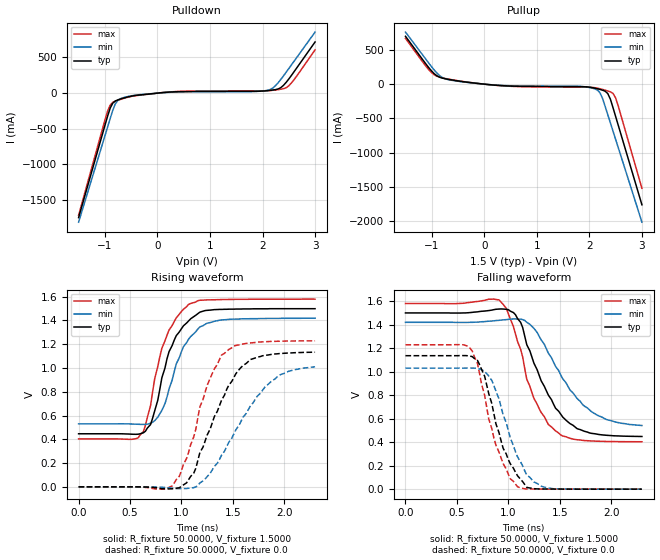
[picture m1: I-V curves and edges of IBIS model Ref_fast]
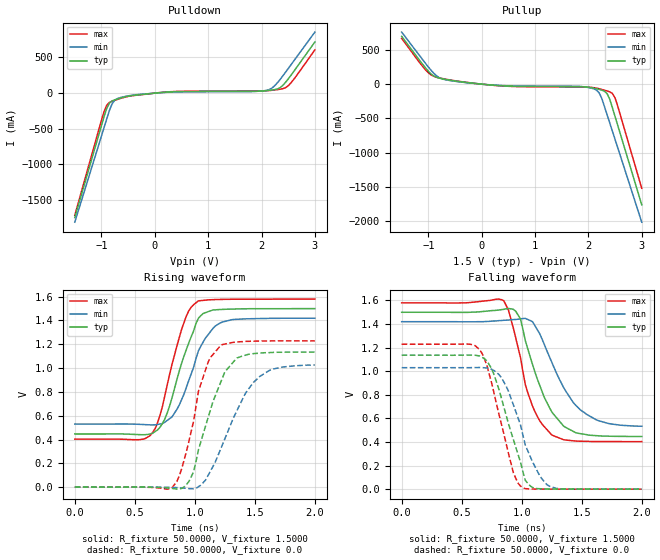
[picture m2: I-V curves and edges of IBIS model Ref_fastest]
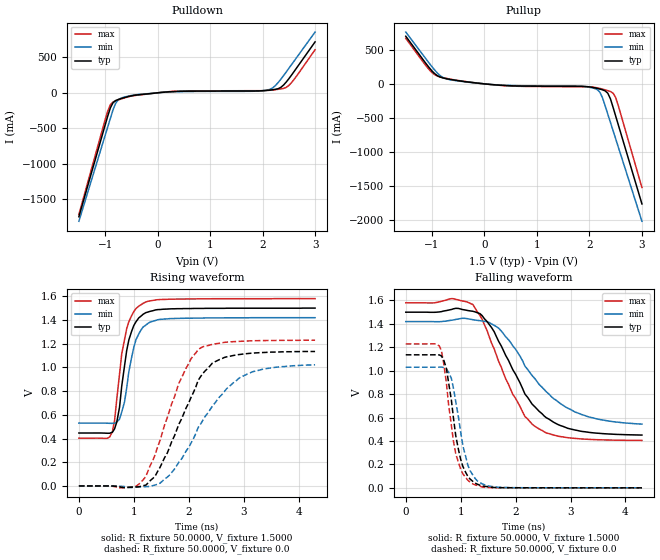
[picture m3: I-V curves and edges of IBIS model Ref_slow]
| Integrated Devices Technolgy, Inc
[IBIS Ver]   4.1
[File name]   9fgu0631.ibs
[File Rev]   1.0
|Rev history   1.0   original revision, 906 LP_HCSL updated for 1.5V operation, IH
[Date]   09 October, 2015
[Disclaimer] Integrated Device Technology, Inc. ("IDT") hereby grants the
   user of this ibis model a non-exclusive, nontransferable
   license to use this ibis model under the following terms. the
   user is granted this license only to use the ibis model and is
   not granted rights to sell, copy (except as needed to run the
   ibis model), rent, lease or sub-license the ibis model in
   whole or in part, or in modified form to anyone. the user may
   modify the ibis model to suit its specific applications, but
   rights to derivative works and such modifications shall belong
   to idt. this ibis model is provided on an as is" basis and idt
   makes absolutely no warranty with respect to the information
   contained herein. idt disclaims and customer waives all
   warranties, express and implied, including warranties of
   merchantability and fitness for a particular purpose. the
   entire risk as to quality and performance is with the user
   accordingly, in no event shall idt be liable for any direct or
   indirect damages, whether in contract or tort, including any
   lost profits or other incidental, consequential, exemplary, or
   punitive damages arising out of the use or application of the
   ibis model. further, idt reserves the right to make changes
   without notice to any product herein to improve reliability,
   function, or design. idt does not convey any license under
   patent rights or any other intellectual property rights,
   including those of third parties. idt is not obligated to
   provide maintenance or support for the licensed ibis model.
[Copyright]   Copyright 2012, Integrated Devices Technolgy, Inc. all rights
   reserved
[Component]   9fgu0631
[Manufacturer] Integrated Device Technology, Inc.
[Package]
|40-VFQFPN
|variable   typ   min   max
R_pkg   81.1m   62.2m   100.0m
L_pkg   6.7nH   4.9nH   8.5nH
C_pkg   0.53pF   0.21pF   0.85pF
[Pin] signal_name  model_name
1   vSS_EN_tri   IN
2   XIN/CLKIN_25   IN
3   X2   NC
4   VDDXTAL1.5   POWER
5   VDDREF1.5   POWER
6   vSADR/REF1.5   REF
7   NC   NC
8   GNDDIG   GND
9   SCLK_3.3   SCIN
10   SDATA_3.3   SCIN
11   VDDDIG1.5   POWER
12   VDDIO   POWER
13   vOE0#   IN
14   DIF0   LP_HCSL
15   DIF0#   LP_HCSL
16   VDD1.5   POWER
17   VDDIO   POWER
18   DIF1   LP_HCSL
19   DIF1#   LP_HCSL
20   NC   NC
21   vOE1#   IN
22   DIF2   LP_HCSL
23   DIF2#   LP_HCSL
24   vOE2#   IN
25   NC   NC
26   VDDA1.5   POWER
27   VDDIO   POWER
28   DIF3   LP_HCSL
29   DIF3#   LP_HCSL
30   vOE3#   IN
31   VDD1.5   POWER
32   VDDIO   POWER
33   DIF4   LP_HCSL
34   DIF4#   LP_HCSL
35   vOE4#   IN
36   DIF5   LP_HCSL
37   DIF5#   LP_HCSL
38   vOE5#   IN
39   VDDIO   POWER
40   ^CKPWRGD_PD   PD
41   ePAD   GND
[Diff Pin]  inv_pin  vdiff tdelay_typ tdelay_min  tdelay_max
14   15   NA   0   0   0
18   19   NA   0   0   0
22   23   NA   0   0   0
28   29   NA   0   0   0
33   34   NA   0   0   0
36   37   NA   0   0   0
[Model Selector] REF
Ref_fast amplitude 1.5, slew rate fast
Ref_fastest amplitude 1.5, slew rate fastest
Ref_slow amplitude 1.5, slew rate slow
Ref_slowest amplitude 1.5, slew rate slowest
[Model Selector] LP_HCSL
lphcsl_0v6_fast amplitude 0.6V, slew rate fast
lphcsl_0v6_slow amplitude 0.6V, slew rate slow
lphcsl_0v7_fast amplitude 0.7V, slew rate fast
lphcsl_0v7_slow amplitude 0.7V, slew rate slow
lphcsl_0v8_fast amplitude 0.8V, slew rate fast
lphcsl_0v8_slow amplitude 0.8V, slew rate slow
lphcsl_0v9_fast amplitude 0.9V, slew rate fast
lphcsl_0v9_slow amplitude 0.9V, slew rate slow
| Models and submodels in the file (15): Ref_fast (Output), Ref_fastest (Output), Ref_slow (Output), Ref_slowest (Output), lphcsl_0v6_fast (Output), lphcsl_0v6_slow (Output), lphcsl_0v7_fast (Output), lphcsl_0v7_slow (Output), lphcsl_0v8_fast (Output), lphcsl_0v8_slow (Output), lphcsl_0v9_fast (Output), lphcsl_0v9_slow (Output), IN (Input), SCIN (Input), PD (Input)
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[Model]  Ref_fast
Model_type Output
Polarity   Non-Inverting
Enable   Active-High
Vmeas =  0.9000V
Cref =   5.0000pF
Rref =   0.0
Vref =   0.9000V
C_comp   1.1000pF   1.0000pF   1.2000pF
[Temperature Range]   25.0000   75.0000   0.0
[Voltage Range]   1.5000V   1.4200V   1.5800V
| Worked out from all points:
|   slope of the pulldown table from 0 to 0.225 V, typ, clamps not added: 15.7 ohm
|   slope of the pullup table from 0 to 0.225 V, typ, clamps not added: 14.4 ohm
|   rising waveform, R_fixture 50.0000, V_fixture 1.5000: 20-80 % time 219ps typ, 227ps min, 214ps max; typ from 0.446 V to 1.5 V
|   rising waveform, R_fixture 50.0000, V_fixture 0.0: 20-80 % time 341ps typ, 434ps min, 263ps max; typ from 0 V to 1.13 V
|   falling waveform, R_fixture 50.0000, V_fixture 1.5000: 20-80 % time 330ps typ, 386ps min, 269ps max; typ from 1.5 V to 0.448 V
|   falling waveform, R_fixture 50.0000, V_fixture 0.0: 20-80 % time 229ps typ, 251ps min, 218ps max; typ from 1.14 V to 0 V
[Pulldown]
|Voltage   I(typ)   I(min)   I(max)
-1.5V     -1.745A    -1.809A    -1.713A
-950mV    -327.8mA   -480.1mA   -255.7mA
-900mV    -212.5mA   -359.3mA   -168.3mA
-850mV    -140.3mA   -241.1mA   -129.4mA
-750mV    -94.02mA   -98.51mA   -100.2mA
-450mV    -36.28mA   -31.57mA   -39.68mA
250mV     15.41mA    12.24mA    17.86mA
1.8V      25.49mA    21.55mA    29.47mA
2.15V     39.17mA    51.36mA    36.57mA
2.35V     77.57mA    193.2mA    55.3mA
2.5V      197.9mA    344.2mA    103.1mA
3V        716.8mA    855.6mA    606.3mA
[Pullup]
|Voltage   I(typ)   I(min)   I(max)
-1.5V     699.4mA    760.9mA    669.2mA
-1V       189.6mA    251.3mA    166.1mA
-900mV    121.4mA    161.2mA    115.6mA
-750mV    80mA       79.09mA    84.43mA
350mV     -22.11mA   -19.15mA   -24.57mA
1.8V      -36.31mA   -32.03mA   -41.75mA
2.15V     -66.71mA   -84.88mA   -58.33mA
2.25V     -87.88mA   -207.1mA   -76.93mA
2.35V     -137.7mA   -445.8mA   -99.43mA
2.45V     -344.5mA   -687.2mA   -135.9mA
2.5V      -473.4mA   -808mA     -201.5mA
3V        -1.763A    -2.017A    -1.522A
[Ramp]
| variable   typ   min   max
dV/dt_r  0.6798/0.3452n   0.6060/0.4303n   0.7374/0.2908n
dV/dt_f  0.6310/0.3319n   0.5270/0.3829n   0.7058/0.2936n
R_load = 50.0000
[Rising Waveform]
R_fixture= 50.0000
V_fixture= 1.5000
V_fixture_min= 1.4200
V_fixture_max= 1.5800
|time   V(typ)   V(min)   V(max)
0s        446.5mV    530.1mV    403.2mV
530ps     442.5mV    528.3mV    400.9mV
630ps     454.6mV    525.2mV    463.7mV
700ps     524.1mV    535.3mV    684.1mV
740ps     638.7mV    557.1mV    908.5mV
810ps     918.1mV    643.4mV    1.166V
950ps     1.272V     1.035V     1.422V
1.07ns    1.396V     1.242V     1.535V
1.37ns    1.493V     1.402V     1.575V
2.3ns     1.499V     1.419V     1.579V
[Rising Waveform]
R_fixture= 50.0000
V_fixture= 0.0
V_fixture_min= 0.0
V_fixture_max= 0.0
|time   V(typ)   V(min)   V(max)
0s        0V         0V         0V
910ps     -16.39mV   -11.25mV   7.954mV
980ps     -7.248mV   -15.17mV   88.84mV
1.14ns    156.1mV    -875uV     484.8mV
1.18ns    289.4mV    33.51mV    674.6mV
1.25ns    435.4mV    85.49mV    853.8mV
1.39ns    727.8mV    265.7mV    1.108V
1.58ns    1.005V     551.8mV    1.198V
1.95ns    1.121V     938.1mV    1.225V
2.3ns     1.133V     1.01V      1.229V
[Falling Waveform]
R_fixture= 50.0000
V_fixture= 1.5000
V_fixture_min= 1.4200
V_fixture_max= 1.5800
|time   V(typ)   V(min)   V(max)
0s        1.5V       1.42V      1.58V
910ps     1.533V     1.437V     1.611V
980ps     1.531V     1.443V     1.54V
1.12ns    1.42V      1.447V     1.191V
1.18ns    1.229V     1.42V      935.1mV
1.28ns    1.018V     1.335V     724.8mV
1.39ns    800.1mV    1.157V     549.9mV
1.56ns    588mV      907.6mV    446.1mV
1.81ns    475.1mV    659.1mV    410.3mV
2.3ns     448.4mV    541.7mV    403.6mV
[Falling Waveform]
R_fixture= 50.0000
V_fixture= 0.0
V_fixture_min= 0.0
V_fixture_max= 0.0
|time   V(typ)   V(min)   V(max)
0s        1.136V     1.03V      1.229V
630ps     1.132V     1.031V     1.198V
720ps     1.061V     1.023V     986.4mV
770ps     961.2mV    1.003V     799.1mV
840ps     728.3mV    925.3mV    515.6mV
950ps     348.1mV    632mV      217.3mV
1.09ns    114mV      275.1mV    20.31mV
1.18ns    14.99mV    120.1mV    1.832mV
1.35ns    1.542mV    17.53mV    713.8uV
2.3ns     16.86uV    43.33uV    1.931uV
[Model]  Ref_fastest
Model_type Output
Polarity   Non-Inverting
Enable   Active-High
Vmeas =  0.9000V
Cref =   5.0000pF
Rref =   0.0
Vref =   0.9000V
C_comp   1.1000pF   1.0000pF   1.2000pF
[Temperature Range]   25.0000   75.0000   0.0
[Voltage Range]   1.5000V   1.4200V   1.5800V
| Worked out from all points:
|   slope of the pulldown table from 0 to 0.225 V, typ, clamps not added: 15.7 ohm
|   slope of the pullup table from 0 to 0.225 V, typ, clamps not added: 14.4 ohm
|   rising waveform, R_fixture 50.0000, V_fixture 1.5000: 20-80 % time 199ps typ, 204ps min, 177ps max; typ from 0.446 V to 1.5 V
|   rising waveform, R_fixture 50.0000, V_fixture 0.0: 20-80 % time 214ps typ, 277ps min, 173ps max; typ from 0 V to 1.14 V
|   falling waveform, R_fixture 50.0000, V_fixture 1.5000: 20-80 % time 225ps typ, 269ps min, 184ps max; typ from 1.5 V to 0.447 V
|   falling waveform, R_fixture 50.0000, V_fixture 0.0: 20-80 % time 201ps typ, 211ps min, 177ps max; typ from 1.14 V to 0 V
[Pulldown]
|Voltage   I(typ)   I(min)   I(max)
-1.5V     -1.745A    -1.809A    -1.713A
-950mV    -327.8mA   -480.1mA   -255.7mA
-900mV    -212.5mA   -359.3mA   -168.3mA
-850mV    -140.3mA   -241.1mA   -129.4mA
-750mV    -94.02mA   -98.51mA   -100.2mA
-450mV    -36.28mA   -31.57mA   -39.68mA
250mV     15.41mA    12.24mA    17.86mA
1.8V      25.49mA    21.55mA    29.47mA
2.15V     39.17mA    51.36mA    36.57mA
2.35V     77.57mA    193.2mA    55.3mA
2.5V      197.9mA    344.2mA    103.1mA
3V        716.8mA    855.6mA    606.3mA
[Pullup]
|Voltage   I(typ)   I(min)   I(max)
-1.5V     699.4mA    760.9mA    669.2mA
-1V       189.6mA    251.3mA    166.1mA
-900mV    121.4mA    161.2mA    115.6mA
-750mV    80mA       79.09mA    84.43mA
350mV     -22.11mA   -19.15mA   -24.57mA
1.8V      -36.31mA   -32.03mA   -41.75mA
2.15V     -66.71mA   -84.88mA   -58.33mA
2.25V     -87.88mA   -207.1mA   -76.93mA
2.35V     -137.7mA   -445.8mA   -99.43mA
2.45V     -344.5mA   -687.2mA   -135.9mA
2.5V      -473.4mA   -808mA     -201.5mA
3V        -1.763A    -2.017A    -1.522A
[Ramp]
| variable   typ   min   max
dV/dt_r  0.6810/0.2229n   0.6156/0.2774n   0.7374/0.1932n
dV/dt_f  0.6319/0.2282n   0.5320/0.2690n   0.7060/0.2043n
R_load = 50.0000
[Rising Waveform]
R_fixture= 50.0000
V_fixture= 1.5000
V_fixture_min= 1.4200
V_fixture_max= 1.5800
|time   V(typ)   V(min)   V(max)
0s        446.5mV    530.1mV    403.2mV
630ps     447mV      523.1mV    434.1mV
690ps     481.3mV    526.5mV    542.2mV
750ps     572.5mV    545.7mV    768mV
850ps     902.3mV    652.2mV    1.183V
950ps     1.213V     897.3mV    1.482V
1.03ns    1.419V     1.145V     1.565V
1.15ns    1.488V     1.332V     1.575V
1.23ns    1.493V     1.387V     1.577V
2ns       1.5V       1.419V     1.58V
[Rising Waveform]
R_fixture= 50.0000
V_fixture= 0.0
V_fixture_min= 0.0
V_fixture_max= 0.0
|time   V(typ)   V(min)   V(max)
0s        0V         0V         0V
810ps     -10.62mV   -2.241mV   -4.352mV
890ps     -10.75mV   -6.644mV   152.2mV
1.01ns    216.9mV    -9.648mV   681.3mV
1.13ns    648.7mV    134.3mV    1.089V
1.25ns    967.4mV    405.7mV    1.202V
1.35ns    1.085V     641.1mV    1.219V
1.49ns    1.122V     882mV      1.226V
1.62ns    1.13V      979.7mV    1.228V
2ns       1.135V     1.026V     1.229V
[Falling Waveform]
R_fixture= 50.0000
V_fixture= 1.5000
V_fixture_min= 1.4200
V_fixture_max= 1.5800
|time   V(typ)   V(min)   V(max)
0s        1.5V       1.42V      1.58V
850ps     1.525V     1.432V     1.599V
890ps     1.532V     1.434V     1.517V
990ps     1.443V     1.444V     1.116V
1.03ns    1.26V      1.448V     888.1mV
1.09ns    1.058V     1.42V      704.3mV
1.25ns    655.5mV    1.078V     460.1mV
1.49ns    470.3mV    670.9mV    406.6mV
1.72ns    449.3mV    557.6mV    403.6mV
2ns       446.8mV    533.3mV    403.3mV
[Falling Waveform]
R_fixture= 50.0000
V_fixture= 0.0
V_fixture_min= 0.0
V_fixture_max= 0.0
|time   V(typ)   V(min)   V(max)
0s        1.136V     1.03V      1.229V
570ps     1.137V     1.03V      1.229V
650ps     1.129V     1.032V     1.183V
750ps     1.021V     1.017V     898.6mV
830ps     775.7mV    947.7mV    555.6mV
930ps     423.1mV    716.8mV    141.6mV
1.01ns    147.3mV    458.1mV    10.69mV
1.09ns    14.41mV    232mV      1.504mV
1.23ns    1.161mV    25.5mV     376.5uV
2ns       -22.42uV   21.58uV    0V
[Model]  Ref_slow
Model_type Output
Polarity   Non-Inverting
Enable   Active-High
Vmeas =  0.9000V
Cref =   5.0000pF
Rref =   0.0
Vref =   0.9000V
C_comp   1.1000pF   1.0000pF   1.2000pF
[Temperature Range]   25.0000   75.0000   0.0
[Voltage Range]   1.5000V   1.4200V   1.5800V
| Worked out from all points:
|   slope of the pulldown table from 0 to 0.225 V, typ, clamps not added: 15.7 ohm
|   slope of the pullup table from 0 to 0.225 V, typ, clamps not added: 14.4 ohm
|   rising waveform, R_fixture 50.0000, V_fixture 1.5000: 20-80 % time 212ps typ, 217ps min, 213ps max; typ from 0.446 V to 1.5 V
|   rising waveform, R_fixture 50.0000, V_fixture 0.0: 20-80 % time 647ps typ, 857ps min, 569ps max; typ from 0 V to 1.13 V
|   falling waveform, R_fixture 50.0000, V_fixture 1.5000: 20-80 % time 763ps typ, 912ps min, 658ps max; typ from 1.5 V to 0.451 V
|   falling waveform, R_fixture 50.0000, V_fixture 0.0: 20-80 % time 234ps typ, 246ps min, 226ps max; typ from 1.14 V to 0 V
[Pulldown]
|Voltage   I(typ)   I(min)   I(max)
-1.5V     -1.745A    -1.809A    -1.713A
-950mV    -327.8mA   -480.1mA   -255.7mA
-900mV    -212.5mA   -359.3mA   -168.3mA
-850mV    -140.3mA   -241.1mA   -129.4mA
-750mV    -94.02mA   -98.51mA   -100.2mA
-450mV    -36.28mA   -31.57mA   -39.68mA
250mV     15.41mA    12.24mA    17.86mA
1.8V      25.49mA    21.55mA    29.47mA
2.15V     39.17mA    51.36mA    36.57mA
2.35V     77.57mA    193.2mA    55.3mA
2.5V      197.9mA    344.2mA    103.1mA
3V        716.8mA    855.6mA    606.3mA
[Pullup]
|Voltage   I(typ)   I(min)   I(max)
-1.5V     699.4mA    760.9mA    669.2mA
-1V       189.6mA    251.3mA    166.1mA
-900mV    121.4mA    161.2mA    115.6mA
-750mV    80mA       79.09mA    84.43mA
350mV     -22.11mA   -19.15mA   -24.57mA
1.8V      -36.31mA   -32.03mA   -41.75mA
2.15V     -66.71mA   -84.88mA   -58.33mA
2.25V     -87.88mA   -207.1mA   -76.93mA
2.35V     -137.7mA   -445.8mA   -99.43mA
2.45V     -344.5mA   -687.2mA   -135.9mA
2.5V      -473.4mA   -808mA     -201.5mA
3V        -1.763A    -2.017A    -1.522A
[Ramp]
| variable   typ   min   max
dV/dt_r  0.6804/0.6793n   0.6132/0.8910n   0.7374/0.5687n
dV/dt_f  0.6296/0.7983n   0.5254/0.9479n   0.7052/0.6762n
R_load = 50.0000
[Rising Waveform]
R_fixture= 50.0000
V_fixture= 1.5000
V_fixture_min= 1.4200
V_fixture_max= 1.5800
|time   V(typ)   V(min)   V(max)
0s        446.5mV    530.1mV    403.2mV
610ps     452.9mV    527.7mV    456.5mV
650ps     482mV      529.1mV    552.8mV
740ps     662.8mV    563.9mV    942.7mV
780ps     841.5mV    623.1mV    1.113V
870ps     1.141V     826mV      1.326V
1ns       1.353V     1.169V     1.47V
1.17ns    1.448V     1.341V     1.54V
1.69ns    1.494V     1.412V     1.575V
4.3ns     1.5V       1.419V     1.58V
[Rising Waveform]
R_fixture= 50.0000
V_fixture= 0.0
V_fixture_min= 0.0
V_fixture_max= 0.0
|time   V(typ)   V(min)   V(max)
0s        0V         0V         0V
960ps     -10.09mV   -13.14mV   -9.522mV
1.17ns    2.233mV    -6.687mV   51.72mV
1.39ns    84.76mV    8.463mV    266.4mV
1.65ns    324.8mV    91.27mV    636.1mV
1.95ns    655.8mV    292.9mV    991.9mV
2.22ns    924.9mV    524.5mV    1.165V
2.43ns    1.036V     672.7mV    1.194V
2.95ns    1.11V      919.4mV    1.22V
4.3ns     1.134V     1.022V     1.229V
[Falling Waveform]
R_fixture= 50.0000
V_fixture= 1.5000
V_fixture_min= 1.4200
V_fixture_max= 1.5800
|time   V(typ)   V(min)   V(max)
0s        1.5V       1.42V      1.58V
830ps     1.523V     1.431V     1.616V
1.22ns    1.508V     1.436V     1.566V
1.39ns    1.471V     1.425V     1.44V
1.69ns    1.252V     1.364V     1.081V
2.17ns    800.7mV    1.039V     608.7mV
2.43ns    652.9mV    882.3mV    502mV
2.74ns    548.1mV    747.4mV    445.3mV
3.08ns    493.8mV    648.1mV    422.1mV
4.3ns     450.7mV    544.3mV    404.7mV
[Falling Waveform]
R_fixture= 50.0000
V_fixture= 0.0
V_fixture_min= 0.0
V_fixture_max= 0.0
|time   V(typ)   V(min)   V(max)
0s        1.136V     1.03V      1.229V
610ps     1.135V     1.031V     1.212V
650ps     1.126V     1.031V     1.169V
740ps     1.02V      1.015V     894.9mV
830ps     751.2mV    934.8mV    534.9mV
910ps     445.7mV    736mV      290.7mV
1.04ns    182.7mV    358.7mV    119.3mV
1.22ns    55.51mV    110.5mV    33.46mV
1.69ns    2.012mV    4.689mV    685uV
4.3ns     21.08uV    30.64uV    -10.67uV
